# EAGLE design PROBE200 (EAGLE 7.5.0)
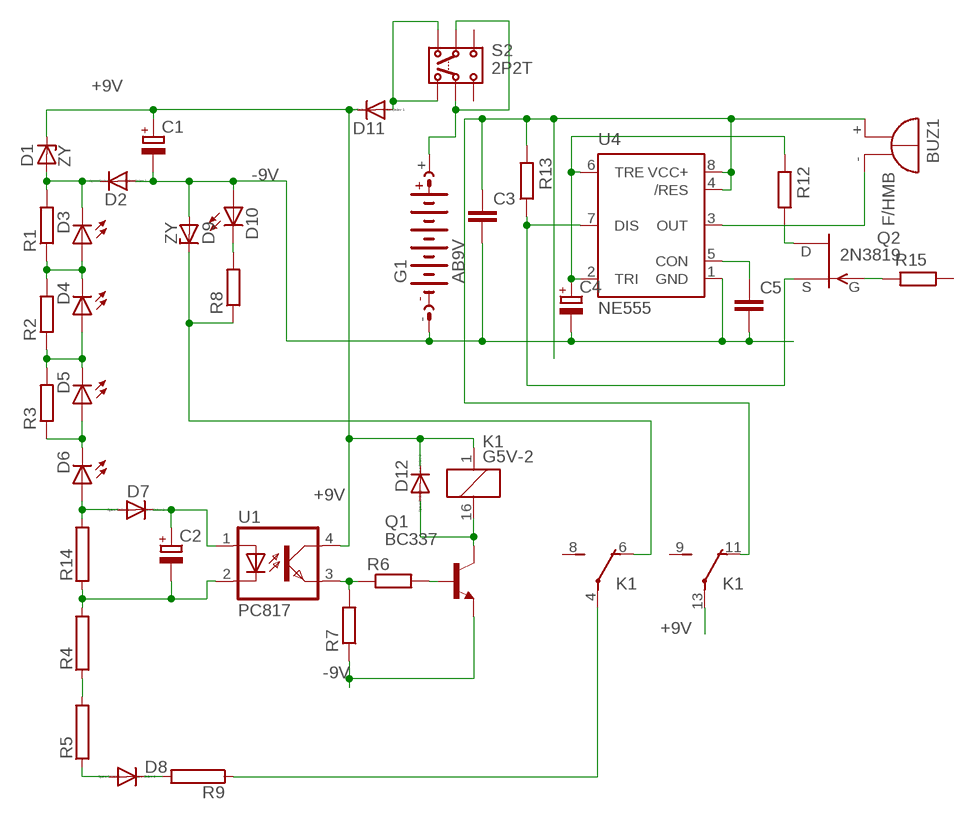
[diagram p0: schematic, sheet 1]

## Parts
BUZ1  F/HMB  [F/HMB]
C1  CPOL-EUE5-10.5  [E5-10,5]
C2  CPOL-EUE5-10.5  [E5-10,5]
C3  C-EUC1206  [C1206]
C4  CPOL-EUE5-10.5  [E5-10,5]
C5  C-EUC1206  [C1206]
D1  ZY  [P1Z12]
D2  1N4004  [DO41-10]
D3  LED5MM  [LED5MM]
D4  LED5MM  [LED5MM]
D5  LED5MM  [LED5MM]
D6  LED5MM  [LED5MM]
D7  1N4004  [DO41-10]
D8  1N4004  [DO41-10]
D9  ZY  [P1Z12]
D10  LED5MM  [LED5MM]
D11  1N4004  [DO41-10]
D12  1N4004  [DO41-10]
G1  AB9V  [AB9V]
K1  G5V-2  [G5V-2]
Q1  BC337  [TO92]
Q2  2N3819  [TO92]
R1  R-EU_0309/12  [0309/12]
R2  R-EU_0309/12  [0309/12]
R3  R-EU_0309/12  [0309/12]
R4  RAC07  [AC07]
R5  RAC07  [AC07]
R6  R-EU_0204/7  [0204/7]
R7  R-EU_0204/7  [0204/7]
R8  R-EU_0309/12  [0309/12]
R9  RAC07  [AC07]
R12  R-EU_0207/10  [0207/10]
R13  R-EU_0207/10  [0207/10]
R14  RAC07  [AC07]
R15  R-EU_0204/7  [0204/7]
S2  2P2T  [2P2T]
U1  PC817  [DIL04]
U4  NE555  [DIL-08]

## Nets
+9V: C1.+ D1.C D11.C D12.C K1.1 K1.13(2:P) U1.4(COL)
-9V: C1.- C3.2 C4.- C5.2 D2.A D9.A D10.A G1.- Q1.1(E) R7.1 U4.1(GND)
N$1: D3.A D4.K(C) R1.1 R2.2
N$2: D6.A D7.A R14.2
N$3: D4.A D5.K(C) R2.1 R3.2
N$4: D5.A D6.K(C) R3.1
N$5: C2.- R4.2 R14.1 U1.2(C)
N$6: R4.1 R5.2
N$7: D8.A R5.1
N$8: D8.C R9.2
N$9: D1.A D2.C D3.K(C) R1.2
N$10: C2.+ D7.C U1.1(A)
N$11: D10.K(C) R8.2
N$12: D12.A K1.16 Q1.3(C)
N$13: Q2.3(S) R13.1 U4.7(DIS)
N$14: D9.C K1.6(1:O) R8.1
N$15: R6.1 R7.2 U1.3(EMIT)
N$16: Q1.2(B) R6.2
N$17: K1.4(1:P) R9.1
N$18: BUZ1.+ C3.1 K1.11(2:O) R13.2 U4.4(/RES) U4.8(VCC+)
N$19: BUZ1.- U4.3(OUT)
N$20: C4.+ R12.2 U4.2(TRI) U4.6(TRE)
N$21: C5.1 U4.5(CON)
N$22: Q2.1(D) R12.1
N$23: D11.A S2.1.1 S2.1.2
N$24: Q2.2(G) R15.2
N$25: G1.+ S2.2.1 S2.2.2
Unconnected: K1.8(1:S) K1.9(2:S) R15.1 S2.3.1 S2.3.2

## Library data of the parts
BUZ1 = buzzer:F/HMB: BUZZER; OC_FARNELL: unknown; OC_NEWARK: unknown
C1 C2 C4 = rcl:CPOL-EU: POLARIZED CAPACITOR, European symbol
C3 C5 = rcl:C-EU: CAPACITOR, European symbol
D1 D9 = diode:ZY: Z DIODE
D2 D7 D8 D11 D12 = diode:1N4004: DIODE
D3-D6 D10 = led:LED: LED
G1 = battery:AB9V: 9-V BATTERY CLIP
K1 = relay:G5V-2: OMRON PCB Relay Source: http://www.omron.com/ecb/products/pdf/en-g5v2.pdf; MPN: G5V-2 5DC; OC_FARNELL: 9949488; OC_NEWARK: 78K5703
Q1 = transistor:BC337: NPN TRANSISTOR
Q2 = transistor-fet:2N3819: N-Channel Junction FET
R1-R3 R6-R8 R12 R13 R15 = rcl:R-EU_: RESISTOR, European symbol
R4 R5 R9 R14 = resistor-power:R: Power Resitor; OC_FARNELL: unknown; OC_NEWARK: unknown
S2 = switch:2P2T: SLIDE SWITCH 2P2T Part No. SS-22F05-G(A)4 Source: CANAL ELECTRONIC CO., LTD .. switsch.pdf
U1 = optocoupler:PC817: SHARP OPTO COUPLER; MPN: PC817X4J000F; OC_FARNELL: 9707727; OC_NEWARK: 97K7059
U4 = st-microelectronics:NE555: General purpose bipolar Timer; MF: Arrow Electronics; MPN: NE555N; OC_FARNELL: 1467742; OC_NEWARK: 89K1486

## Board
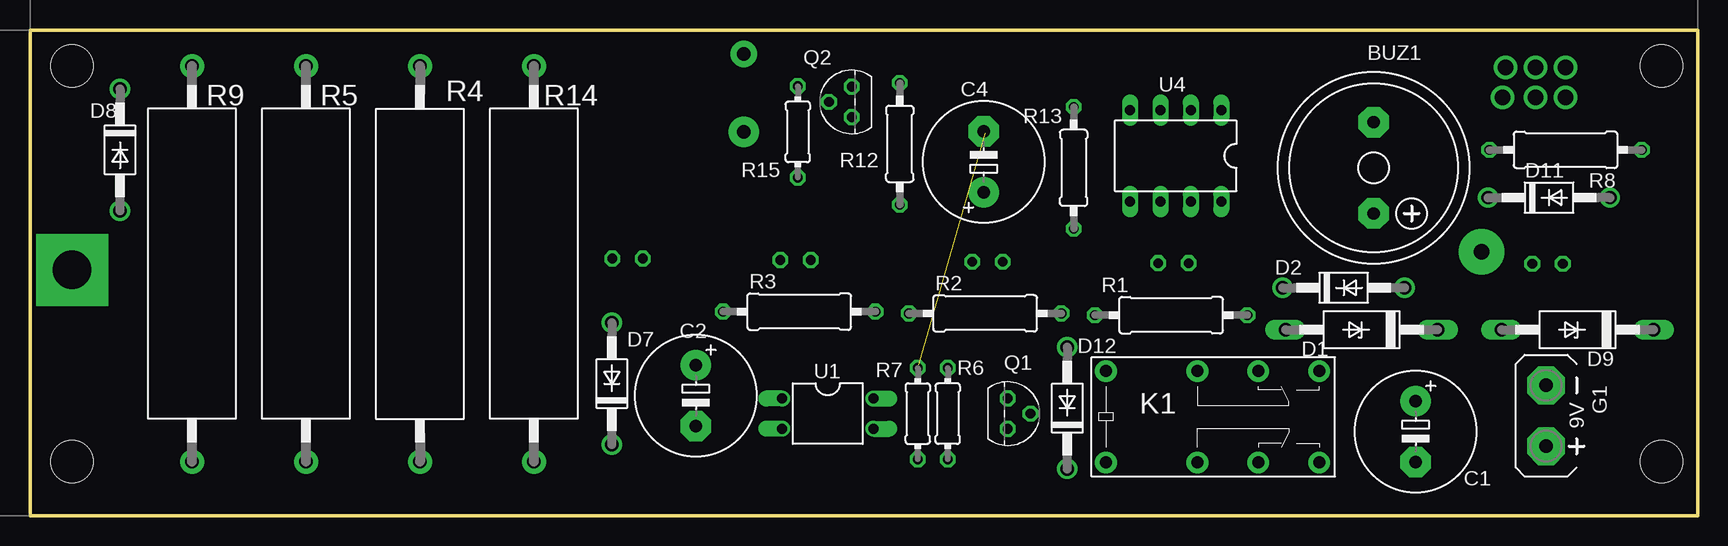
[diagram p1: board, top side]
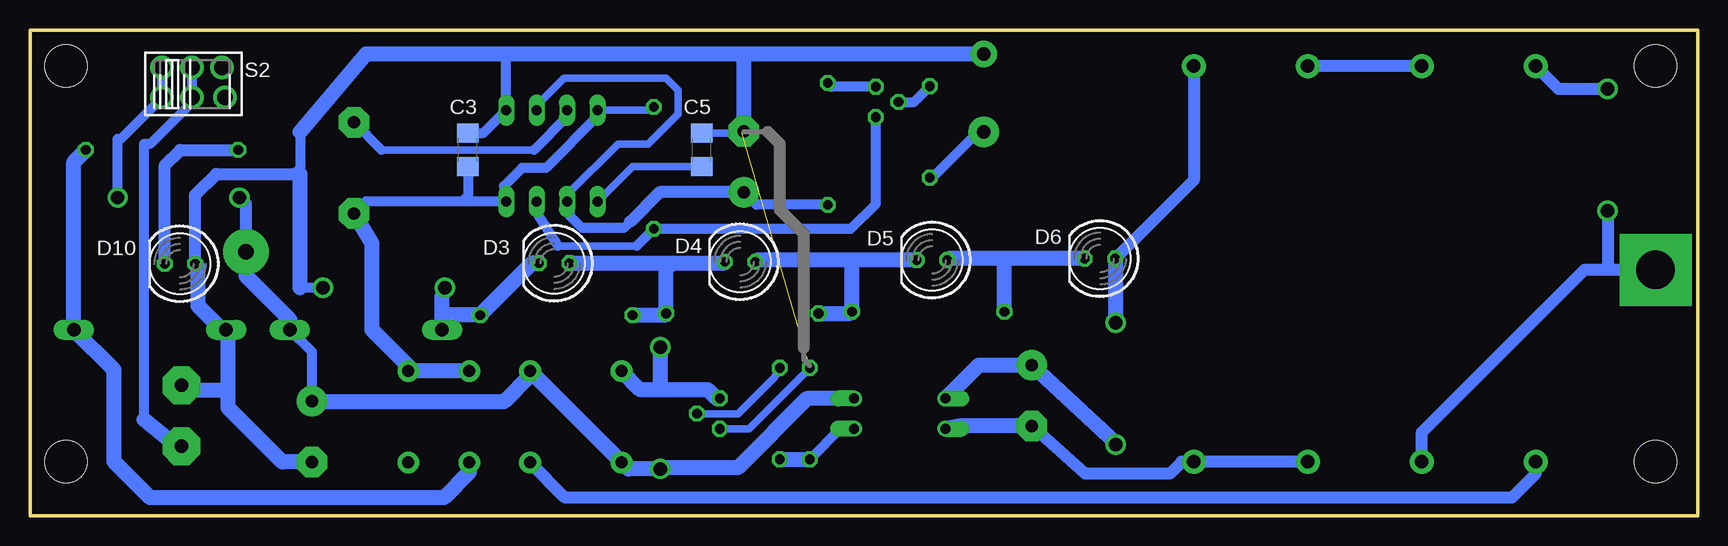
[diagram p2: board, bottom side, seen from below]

Size 139 x 40.5 mm. Coordinates in mm from the lower left corner, seen from the top.
Outline: 0,0 0,40.5 139,40.5 139,0 0,0
Copper layers (1*16): Top 0.035mm / dielectric 1.5mm / Bottom 0.035mm
Design rules "default": minimum track width 10mil, minimum drill 24mil, track to track 8mil, track to pad 8mil, pad to pad 8mil, via to via 8mil, smd to smd 8mil, copper to edge 40mil, drill to drill 8mil, minimum pad ring 10mil, minimum via ring 8mil, stop-mask expansion 4mil, vias tented up to drill 0mil, thermal gap 10mil
Holes 3.5 mm at 3.5,37.5 3.5,4.5 136,4.5 136,37.5

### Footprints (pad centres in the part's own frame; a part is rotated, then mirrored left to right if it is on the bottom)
F/HMB = drill 1.016 pad 2.54 octagon: + 3.81,0; - -3.81,0
E5-10,5 = drill 1.016 pad 2.54: + -2.54,0 | drill 1.016 pad 2.54 octagon: - 2.54,0
C1206 = smd 1.6 x 1.8: 1 -1.4,0; 2 1.4,0
P1Z12 = drill 1.118 long: A 6.35,0; C -6.35,0
DO41-10 = drill 1.118: A 5.08,0; C -5.08,0
LED5MM = drill 0.813 octagon: A -1.27,0; K 1.27,0
AB9V = drill 1.118 pad 3.15 octagon: + 0,2.54; - 0,-2.54
G5V-2 = drill 1 pad 1.8: 1 -8.89,-3.81; 4 -1.27,-3.81; 6 3.81,-3.81; 8 8.89,-3.81; 9 8.89,3.81; 11 3.81,3.81; 13 -1.27,3.81; 16 -8.89,3.81
TO92 = drill 0.813 octagon: 1 1.27,0; 2 0,1.905; 3 -1.27,0
0309/12 = drill 0.813 octagon: 1 -6.35,0; 2 6.35,0
AC07 = drill 1.1 pad 2: 1 -16.5,0; 2 16.5,0
0204/7 = drill 0.813 octagon: 1 -3.81,0; 2 3.81,0
0207/10 = drill 0.813 octagon: 1 -5.08,0; 2 5.08,0
2P2T = drill 1.3 pad 1.93: 1.1 -2.492,1.38; 1.2 -2.492,-1.126; 2.1 0,1.38; 2.2 0,-1.126; 3.1 2.492,1.38; 3.2 2.746,-1.126
DIL04 = drill 0.813 offset: 1 -1.27,-3.81; 2 1.27,-3.81; 3 1.27,3.81; 4 -1.27,3.81
DIL-08 = drill 0.813 long: 1 -3.81,-3.81; 2 -1.27,-3.81; 3 1.27,-3.81; 4 3.81,-3.81; 5 3.81,3.81; 6 1.27,3.81; 7 -1.27,3.81; 8 -3.81,3.81

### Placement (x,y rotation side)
BUZ1  112,29 270 top
C1  115.5,7 270 top
C2  55.5,10 270 top
C3  102.5,30.5 90 bottom
C4  79.5,29.5 90 top
C5  83,30.5 90 bottom
D1  111,15.5 180 top
D2  109.5,19 0 top
D3  95.31,21.05 180 bottom
D4  79.81,21.17 180 bottom
D5  63.81,21.31 180 bottom
D6  49.81,21.43 180 bottom
D7  48.5,11 90 top
D8  7.5,30.5 270 top
D9  129,15.5 180 top
D10  126.5,21 180 bottom
D11  126.62,26.52 0 top
D12  86.46,8.96 90 top
G1  126.38,8.32 180 top
K1  98.58,8.24 0 top
Q1  81.5,8.5 270 top
Q2  68.5,34.5 90 top
R1  95.12,16.71 0 top
R2  79.62,16.86 0 top
R3  64.12,17.01 0 top
R4  32.5,21 270 top
R5  23,21 90 top
R6  76.5,8.5 90 top
R7  74,8.5 270 top
R8  128,30.5 180 top
R9  13.5,21 90 top
R12  72.5,31 270 top
R13  87,29 90 top
R14  42,21 90 top
R15  64,32 90 top
S2  125.5,36 0 bottom
U1  66.5,8.5 270 top
U4  95.5,30 180 top

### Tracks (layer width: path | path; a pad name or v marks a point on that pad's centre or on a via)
+9V  (via drill 1.3 pad 3.81)
  Bottom 0.813: C1.+ 115.5,13.65 D1.C
  Bottom 1.016: D1.C 117.35,15.85 | 120.5,21.5 v121,22 121,25.98 D11.C
  Bottom 1.27: 89.64,4.38 K1.1 | K1.1 K1.13 97.31,11.69 99.5,9.5 114.46,9.5 C1.+ | K1.1 89.14,3.88 D12.C 86.34,4 80,4 74.23,9.77 U1.4 | 117.35,15.85 117.35,16.35 121,20 v121,22
-9V  (via drill 1.1 pad 2.18)  (1 unrouted)
  Bottom 0.61: Q1.1 79.08,7.23 R7.1 | C5.2 79.64,31.9
  Bottom 0.813: D2.A 116.5,19 | 116.5,32 116.5,29 117,28.5 | 99,38.5 99.31,38.19 U4.1 101.22,31.9 C3.2
  Bottom 1.016: D10.A 125.23,26.77 123.5,28.5 117,28.5 116.5,28.5
  Bottom 1.27: 116.5,19 116.5,28.5 | 79.5,38.5 99,38.5 111,38.5 116.5,32 | G1.- 126.24,10.5 122.5,10.5 | C1.- 117.96,4.46 122.5,9 122.5,10.5 | 122.5,10.5 122.5,15.35 D9.A 123,15.5 125,17.5 125,20.77 D10.A | v59.5,38.5 79.5,38.5 | 79.5,38.5 C4.- 79.64,31.9
N$1
  Bottom 1.27: D3.A 85.5,21.05 | 85.5,21.05 81.2,21.05 D4.K | R1.1 86.12,16.71 R2.2 85.97,20.58 85.5,21.05
N$2
  Bottom 1.016: R14.2 42,27.97 D6.A
  Bottom 1.27: D7.A 48.5,21.39 D6.A
N$3
  Bottom 1.27: D5.K 70.5,21.31 | 70.5,21.31 78.4,21.31 D4.A | 70.5,21.31 70.47,21.28 R3.2 70.62,16.86 R2.1
N$4
  Bottom 1.27: D6.K 58,21.43 | 58,21.43 62.42,21.43 D5.A | R3.1 57.77,21.2 58,21.43
N$5
  Bottom 1.016: R4.2 R14.1 43,4.5 44,3.5 51.04,3.5 C2.-
  Bottom 1.27: C2.- 61.46,7.46 U1.2
N$6
  Bottom 1.016: R5.2 R4.1
N$7  (via drill 3.2 pad 6)
  Bottom 1.016: R5.1 23,6.92 9.42,20.5 7.5,20.5 | v3.5,20.5 7.5,20.5 | D8.A 7.5,20.5
N$8
  Bottom 1.016: D8.C 11.58,35.58 R9.2
N$9
  Bottom 1.27: D1.A 104.65,17 | 104.65,17 104.65,18.27 D2.C | 104.65,17 104.36,16.71 R1.2 97.13,21.05 D3.K
N$10
  Bottom 1.27: D7.C 48.5,6.04 C2.+ 59.92,12.54 U1.1
N$11
  Bottom 1.016: D10.K 127.77,29.23 126.5,30.5 R8.2
N$12
  Bottom 1.27: Q1.3 81.77,9.77 82.5,10.5 86.5,10.5 | 86.5,10.5 88.14,10.5 K1.16 | D12.A 86.46,10.54 86.5,10.5
N$13
  Bottom 0.61: 95,22.5 88.42,22.5
  Bottom 0.813: U4.7 96.77,25.27 95,22.5 | 88.42,22.5 R13.1 70.58,23.92 68.5,26 Q2.3
N$14
  Bottom 1.27: K1.6 102.39,3.61 104.5,1.5 129,1.5 132,4.5 132,12.15 D9.C 135.35,29.5 R8.1
N$15
  Bottom 0.813: U1.3 71.46,7.23 R7.2
  Bottom 1.27: R6.1 R7.2
N$16
  Bottom 0.61: R6.2 77,11.5 80,8.5 Q1.2
N$17
  Bottom 1.016: R9.1 13.5,3.5 15.5,1.5 94.38,1.5 K1.4
N$18
  Bottom 0.61: U4.4 87.27,33.81 R13.2
  Bottom 0.813: 103,26.19 U4.8 99.5,26.38 99.5,27.5 98,29 96,29 91.69,33.31 U4.4 | 103,26.19 111,26.19 BUZ1.+ | C3.1 102.5,26.69 103,26.19
  Bottom 1.27: K1.11 107.05,12.05 110.5,15.5 110.5,22.69 BUZ1.+
N$19
  Bottom 0.61: 97,30.5 109.69,30.5
  Bottom 0.813: U4.3 94.23,33.27 97,30.5 | 109.69,30.5 BUZ1.-
N$20
  Bottom 0.61: U4.6 94.23,26.77 90,31 87.5,31 85,33.5 85,35.5 86,36.5 94.5,36.5 96.5,34.5 96.5,34.08 U4.2
  Bottom 0.813: 89,24.5 89.5,24 93,24 94,25 94,25.96 U4.6 | R12.2 78.46,25.92 C4.+
  Bottom 1.016: C4.+ 86.54,26.96 89,24.5
N$21
  Bottom 0.61: C5.1 88.78,29.1 U4.5
N$22
  Bottom 0.813: Q2.1 72.19,35.77 R12.1
N$23
  Bottom 0.813: D11.A 131.7,31.41 131.45,31.41 S2.1.2 S2.1.1
N$24
  Bottom 0.813: Q2.2 65.31,34.5 R15.2
N$25
  Bottom 0.813: 129.5,8 129.5,31 129,31 125.5,34.5 S2.2.2 S2.2.1
  Bottom 1.27: G1.+ 126.78,5.78 129.5,8
N$26  (via drill 1.1 pad 2.54)
  Bottom 0.813: v59.5,32 60,32 64,28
